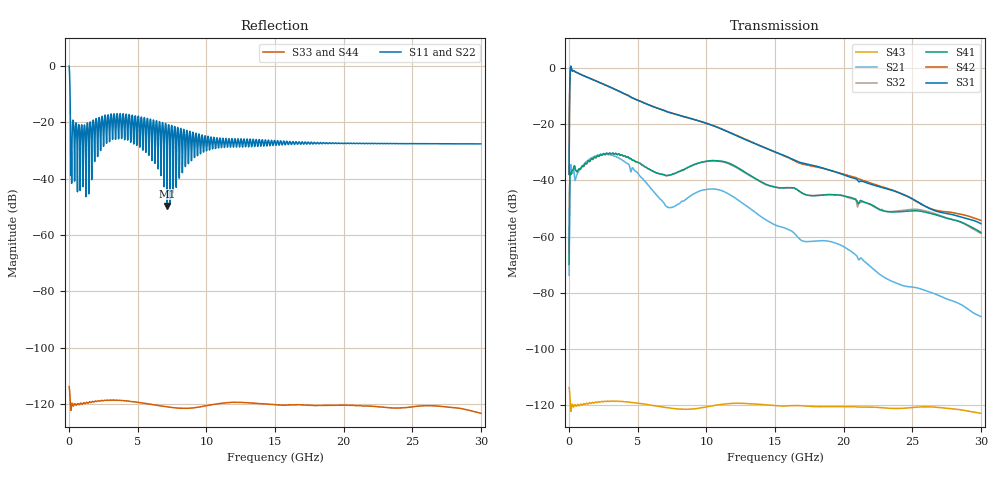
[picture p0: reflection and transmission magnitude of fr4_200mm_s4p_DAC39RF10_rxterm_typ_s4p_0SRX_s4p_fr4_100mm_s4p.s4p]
! Touchstone generated by fitter/viewer
# HZ S  RI R 5.000000e+01
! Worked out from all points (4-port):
!   3899 points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, 7.694 MHz to 30 GHz, reference 50 ohm
!   strongest paths, dB at 7.694 MHz, 7.502 GHz, 15 GHz, 22.51 GHz, 30 GHz:
!     S31: -37.9, -16.0, -29.8, -42.1, -55.4
!     S42: -37.8, -16.0, -29.9, -41.8, -54.3
!     S41: -69.7, -37.9, -42.3, -50.0, -58.5
!     S32: -70.2, -37.9, -42.4, -50.2, -58.9
!     S21: -73.8, -49.6, -55.8, -73.0, -88.5
!     S43: -113.8, -121.2, -120.2, -120.9, -123.0
!   lowest |S11| = -49.7 dB at 7.148 GHz (marker M1), VSWR 1.01, Z = 50.3 - j0.103 ohm
!   |S11| at or under -10 dB: 76.95 MHz to end of sweep
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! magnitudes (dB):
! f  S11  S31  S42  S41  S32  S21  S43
! 7.694 MHz  -0.1  -37.9  -37.8  -69.7  -70.2  -73.8  -113.8
! 223.1 MHz  -25.8  -0.9  -0.9  -36.5  -36.4  -37.5  -119.7
! 2.17 GHz  -18.8  -5.0  -5.0  -31.4  -31.5  -31.0  -118.8
! 7.148 GHz  -49.7  -15.5  -15.5  -38.2  -38.3  -49.4  -121.0
! 10.97 GHz  -25.9  -21.4  -21.3  -33.1  -33.3  -43.4  -119.9
! 23.98 GHz  -27.6  -44.3  -44.3  -51.2  -50.8  -76.8  -121.2
! 30 GHz  -27.7  -55.4  -54.3  -58.5  -58.9  -88.5  -123.0
